(* Logix 5000 AddOnInstructionDefinition export; software revision 16.00 *)

ADD_ON_INSTRUCTION AMCI_ANG1E_Enable_Driver   (* revision 1.0, vendor AMCI *)
VAR_IN_OUT
   AMCI_ANG1E_output_data : INT[10]; {required}
END_VAR
VAR
   command_data_block : INT[10];
        [0]   // Command Bits MSW
        [1]   // Command Bits LSW
        [2]   // Upper Target Position
        [3]   // Lower Target Position
        [4]   // Upper Programmed Speed
        [5]   // Lower Programmed Speed
END_VAR

ROUTINE Logic   (* ladder *)
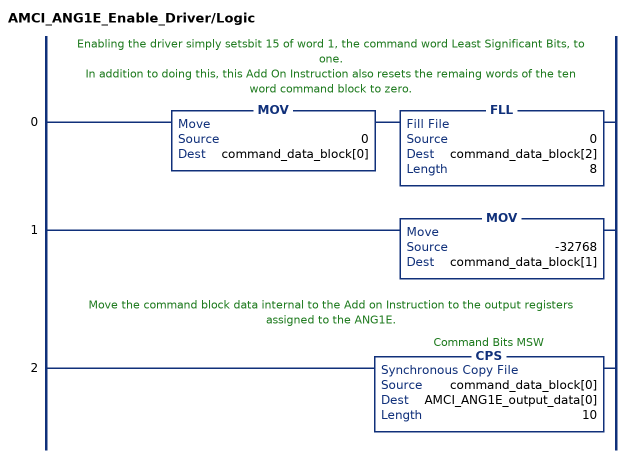
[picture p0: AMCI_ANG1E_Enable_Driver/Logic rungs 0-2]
   // Enabling the driver simply setsbit 15 of word 1, the command word Least Significant Bits, to one.
   // In addition to doing this, this Add On Instruction also resets the remaing words of the ten word command block to zero.
   0: MOV(0,command_data_block[0])FLL(0,command_data_block[2],8);
   1: MOV(-32768,command_data_block[1]);
   // Move the command block data internal to the Add on Instruction to the output registers assigned to the ANG1E.
   2: CPS(command_data_block[0],AMCI_ANG1E_output_data[0],10);
END_ROUTINE
END_ADD_ON_INSTRUCTION
